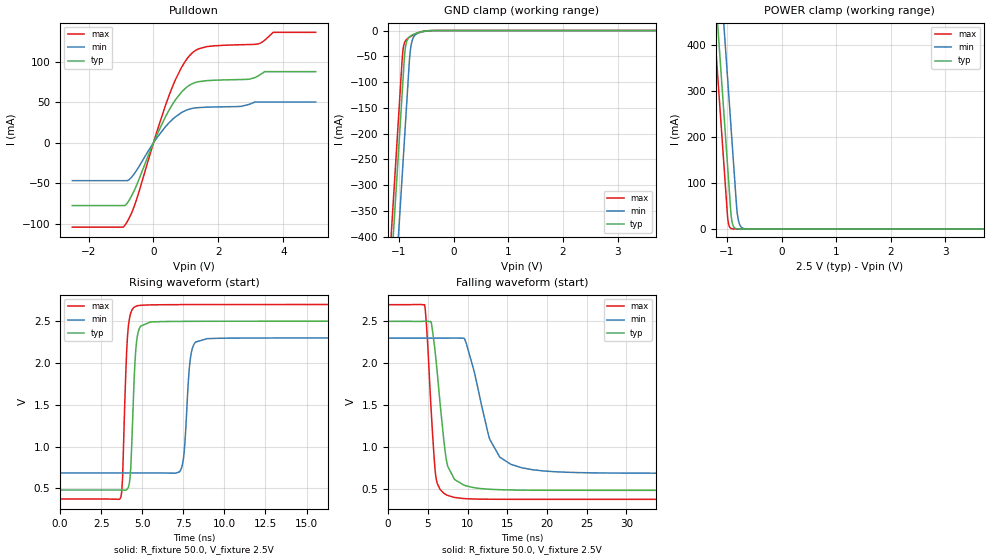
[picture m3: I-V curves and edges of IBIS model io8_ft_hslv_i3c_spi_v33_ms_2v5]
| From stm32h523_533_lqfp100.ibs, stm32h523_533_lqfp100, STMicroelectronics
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[Model]   io8_ft_hslv_i3c_spi_v33_ms_2v5
Model_type I/O_open_drain
Polarity   Non-Inverting
Enable   Active-Low
| CAP_THRESHOLD on pad IOFT is "UDTCAPC" :
| Rising=20.0% of vddiom   Falling=80.0% of vddiom
| C_comp min and max val. don't necessarily correlate with the min and max pvt
| but are the smallest and greatest pad capacitance found.
| var   typ   min   max
C_comp   3.86841pF  3.83550pF  3.96274pF
|C_comp_pulldown   3.86841pF  3.83550pF  3.96274pF
Vinl = 1.15V
Vinh = 1.35V
Vmeas = 1.25V   | Reference voltage for timing measurements
Cref  = 50.0pF   | Timing specification test load capacitance value
Rref  = 1.0MOhm   | Timing specification test load resistance value
Vref  = 1.375V   | Timing specification test load voltage
[Model Spec]
| TIME_THRESHOLD on pin ZII2CV11 is "CMOS" :
| Rising=40.0% of vdd   Falling=60.0% of vdd
Vinl 978.80000mV 906.80000mV 1.05480V
Vinh 1.39920V 1.29220V 1.48720V
| variable   typ   min   max
[Temperature Range] 25.0 125.0 -40.0
| variable   typ   min   max
[Voltage Range] 2.5V 2.3V 2.7V
| variable   typ   min   max
[POWER Clamp Reference] 2.5V 2.3V 2.7V
| variable   typ   min   max
[GND Clamp Reference] 0V 0V 0V
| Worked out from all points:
|   slope of the pulldown table from 0 to 0.375 V, typ, clamps not added: 11.5 ohm
|   GND clamp passes 1 mA (typ) near -0.52 V on its own axis
|   POWER clamp passes 1 mA (typ) near -0.84 V on its own axis
|   rising waveform, R_fixture 50.0, V_fixture 2.5V: 20-80 % time 253ps typ, 304ps min, 242ps max; typ from 0.481 V to 2.5 V
|   falling waveform, R_fixture 50.0, V_fixture 2.5V: 20-80 % time 1.3ns typ, 2.67ns min, 844ps max; typ from 2.5 V to 0.481 V
[POWER Clamp]
-2.5V     2.708A     2.899A     2.597A
-1.23V    548.8mA    740.2mA    437.5mA
-1.16V    429.8mA    621.2mA    318.5mA
-1.12V    361.8mA    553.2mA    250.5mA
-1.03V    208.8mA    400.2mA    97.53mA
-980mV    123.8mA    315.2mA    17.95mA
-920mV    26.3mA     213.2mA    906uA
-880mV    5.543mA    145.2mA    123.7uA
-810mV    363.5uA    33.6mA     3.797uA
-770mV    76.62uA    10.47mA    518.8nA
-700mV    5.026uA    1.361mA    16.09nA
5V        0A         0A         0A
[GND Clamp]
-2.5V     -2.77A     -2.931A    -2.704A
-1.21V    -576.8mA   -738.1mA   -511.3mA
-950mV    -134.8mA   -296.1mA   -69.34mA
-920mV    -83.82mA   -245.1mA   -32.48mA
-900mV    -50.56mA   -211.1mA   -24.02mA
-880mV    -31.31mA   -177.1mA   -19.85mA
-850mV    -18.7mA    -126.1mA   -16.34mA
-800mV    -11.46mA   -46.18mA   -12.45mA
-750mV    -8.203mA   -16.63mA   -9.325mA
-650mV    -4.063mA   -4.987mA   -4.427mA
-360mV    -35.05uA   -165.1uA   -9.564uA
5V        7.96nA     1.282uA    294pA
| variable   typ   min   max
[Pullup Reference] 2.5V 2.3V 2.7V
| variable   typ   min   max
[Pulldown Reference] 0V 0V 0V
[Pulldown]
-2.5V     -77.63mA   -46.85mA   -104.3mA
-870mV    -77.24mA   -46.85mA   -101.4mA
-550mV    -55.3mA    -35.88mA   -73.72mA
90mV      8.401mA    5.299mA    11.79mA
610mV     49.03mA    29.76mA    71.69mA
870mV     62.92mA    37.48mA    93.62mA
1.23V     73.63mA    42.72mA    112.2mA
1.64V     76.78mA    44.01mA    118.8mA
2.7V      78.15mA    44.99mA    121.2mA
3.22V     82.58mA    50.35mA    122.2mA
3.69V     87.93mA    50.35mA    136.5mA
5V        87.93mA    50.35mA    136.5mA
[Ramp]
dV/dt_r 1.21162V/248.59481ps 969.21667mV/300.5838ps 1.39626V/238.23841ps
dV/dt_f 1.21165V/1.30212ns 969.26057mV/2.47971ns 1.39628V/843.28466ps
R_load = 50.0
| Removed startup time: 0s 0s 0s  .
| Removed end time: 33.7ns.
[Rising Waveform]
R_fixture   = 50.0
V_fixture   = 2.5V
V_fixture_min = 2.3V
V_fixture_max = 2.7V
0s        480.6mV    684.6mV    372.9mV
3.7ns     480.4mV    684.6mV    399mV
3.8ns     479.4mV    684.6mV    623.6mV
4.1ns     493.7mV    684.6mV    2.319V
4.3ns     750.8mV    684.6mV    2.6V
4.65ns    2.252V     684.6mV    2.681V
7.35ns    2.498V     725.2mV    2.699V
8ns       2.498V     2.138V     2.699V
8.95ns    2.499V     2.291V     2.7V
33.7ns    2.5V       2.3V       2.7V
| Removed startup time: 0s 0s 0s  .
| Removed end time: 68.75ns.
[Falling Waveform]
R_fixture   = 50.0
V_fixture   = 2.5V
V_fixture_min = 2.3V
V_fixture_max = 2.7V
0s        2.5V       2.3V       2.7V
4.6ns     2.501V     2.3V       2.698V
4.9ns     2.501V     2.3V       2.359V
5.4ns     2.496V     2.3V       1.476V
6ns       2.069V     2.3V       656mV
7.5ns     769.4mV    2.3V       419.8mV
9.65ns    538.9mV    2.287V     381.5mV
12.8ns    493.1mV    1.09V      374mV
16.85ns   482.9mV    749.3mV    373mV
68.75ns   480.6mV    684.6mV    372.9mV
